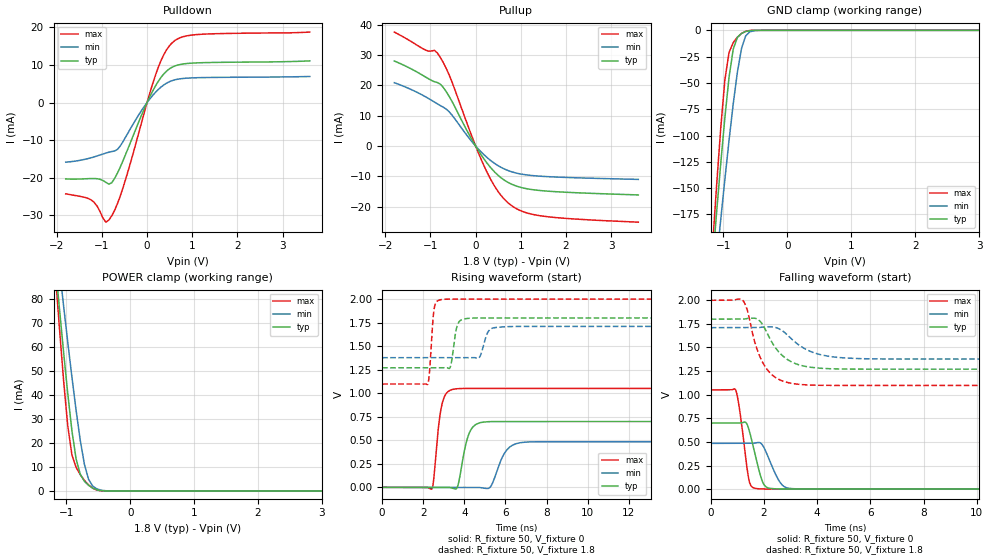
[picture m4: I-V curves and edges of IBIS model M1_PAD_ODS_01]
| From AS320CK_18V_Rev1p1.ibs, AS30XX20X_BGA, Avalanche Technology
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[Model] M1_PAD_ODS_01
Model_type I/O
Enable   Active-High
Vinl  =  0.63
Vinh  =  1.17
Vmeas =  0.9
Cref  =  30e-12
| Capacitance  typ   min   max
C_comp   1.624629e-12   1.520611e-12   1.744819e-12
| Variables   typ   min   max
[GND Clamp Reference]   0   0   0
[POWER Clamp Reference]   1.8   1.71   2
[Pulldown Reference]   0   0   0
[Pullup Reference]   1.8   1.71   2
[Temperature Range]   25   125   -40
[Voltage Range]   1.8   1.71   2
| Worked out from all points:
|   slope of the pulldown table from 0 to 0.27 V, typ, clamps not added: 44.9 ohm
|   slope of the pullup table from 0 to 0.27 V, typ, clamps not added: 45.3 ohm
|   GND clamp passes 1 mA (typ) near -0.64 V on its own axis
|   POWER clamp passes 1 mA (typ) near -0.57 V on its own axis
|   falling waveform, R_fixture 50, V_fixture 0: 20-80 % time 369ps typ, 461ps min, 285ps max; typ from 0.7 V to 0 V
|   falling waveform, R_fixture 50, V_fixture 1.8: 20-80 % time 819ps typ, 1.04ns min, 647ps max; typ from 1.8 V to 1.27 V
|   rising waveform, R_fixture 50, V_fixture 0: 20-80 % time 407ps typ, 569ps min, 308ps max; typ from 0 V to 0.7 V
|   rising waveform, R_fixture 50, V_fixture 1.8: 20-80 % time 214ps typ, 282ps min, 165ps max; typ from 1.27 V to 1.8 V
[GND Clamp]
| Voltage   I(typ)   I(min)   I(max)
-1.8V     -720.4mA   -670.5mA   -825.2mA
-1.173V   -222.3mA   -260.3mA   -207.5mA
-1.108V   -173.8mA   -219.8mA   -148.3mA
-1.043V   -126.9mA   -180.1mA   -93.11mA
-977.6mV  -83.02mA   -141.5mA   -47.01mA
-912.4mV  -44.68mA   -104.6mA   -21.04mA
-847.2mV  -17.95mA   -70.1mA    -11.75mA
-782.1mV  -6.736mA   -39.85mA   -6.526mA
-716.9mV  -2.917mA   -17.13mA   -2.96mA
-651.7mV  -1.107mA   -5.246mA   -907.6uA
-456.2mV  -3.886uA   -74.14uA   -373.5nA
3.6V      0A         0A         0A
[POWER Clamp]
| Voltage   I(typ)   I(min)   I(max)
-1.8V     287.1mA    268.3mA    329.6mA
-1.173V   94.89mA    108.5mA    91.02mA
-1.108V   76.1mA     92.66mA    67.97mA
-1.043V   57.9mA     77.16mA    46.14mA
-977.6mV  40.62mA    62.05mA    27.14mA
-912.4mV  25.13mA    47.46mA    15.06mA
-847.2mV  13.38mA    33.64mA    9.853mA
-716.9mV  4.014mA    11.09mA    4.394mA
-651.7mV  2.34mA     4.821mA    2.483mA
-586.6mV  1.18mA     2.003mA    1.113mA
-325.9mV  1.153uA    19.85uA    110.1nA
3.6V      0A         0A         0A
[Pulldown]
| Voltage   I(typ)   I(min)   I(max)
-1.8V     -20.29mA   -15.84mA   -24.25mA
-1.238V   -20.19mA   -14.67mA   -25.87mA
-912.4mV  -21.19mA   -13.43mA   -31.79mA
-847.2mV  -21.68mA   -13.2mA    -31.24mA
-716.9mV  -20.15mA   -12.86mA   -28.61mA
-521.4mV  -15.14mA   -10.15mA   -22.2mA
-65.17mV  -1.742mA   -1.091mA   -2.802mA
248.3mV   5.63mA     3.46mA     9.353mA
434.5mV   8.383mA    5.171mA    14.07mA
620.7mV   9.735mA    6.051mA    16.51mA
1.179V    10.57mA    6.614mA    18.12mA
3.6V      11.06mA    6.923mA    18.71mA
[Pullup]
| Voltage   I(typ)   I(min)   I(max)
-1.8V     28.07mA    20.9mA     37.6mA
-1.108V   22.77mA    16.25mA    31.67mA
-912.4mV  21.23mA    14.53mA    31.58mA
-782.1mV  20.42mA    13.35mA    29.27mA
-586.6mV  16.4mA     11.32mA    23.49mA
-65.17mV  1.669mA    1.14mA     2.505mA
248.3mV   -5.556mA   -3.722mA   -8.519mA
496.6mV   -9.653mA   -6.467mA   -14.99mA
744.8mV   -12.21mA   -8.229mA   -19.08mA
1.055V    -13.85mA   -9.372mA   -21.68mA
1.49V     -14.76mA   -10.01mA   -23.13mA
3.6V      -16.13mA   -11mA      -25.12mA
[Ramp]
dV/dt_r   0.419845/0.40709n  0.290904/0.569117n  0.630672/0.308383n
dV/dt_f   0.317972/0.818691n  0.199636/1.04487n  0.541445/0.646878n
R_load = 50
[Falling Waveform]
R_fixture = 50
V_fixture = 0
V_fixture_min = 0
V_fixture_max = 0
| Time   V(typ)   V(min)   V(max)
0s        699.7mV    484.8mV    1.051V
936.6ps   700.2mV    485.3mV    1.051V
1.089ns   700.3mV    485.4mV    839.3mV
1.43ns    639mV      485.6mV    108.6mV
1.732ns   294.8mV    491.4mV    6.152mV
1.952ns   76.13mV    465.2mV    2.032mV
2.096ns   21.34mV    384.1mV    1.262mV
2.616ns   1.831mV    69mV       474.1uV
3.058ns   724uV      5.937mV    463.2uV
21.88ns   1.404nV    117.1nV    -317.4nV
[Falling Waveform]
R_fixture = 50
V_fixture = 1.8
V_fixture_min = 1.71
V_fixture_max = 2
| Time   V(typ)   V(min)   V(max)
0s        1.8V       1.71V      2V
1.173ns   1.801V     1.71V      2.008V
1.362ns   1.807V     1.711V     1.909V
1.709ns   1.807V     1.711V     1.511V
2.045ns   1.695V     1.717V     1.297V
2.543ns   1.458V     1.701V     1.165V
3.19ns    1.329V     1.553V     1.114V
4.145ns   1.28V      1.423V     1.1V
5.594ns   1.271V     1.382V     1.098V
21.88ns   1.27V      1.377V     1.098V
[Rising Waveform]
R_fixture = 50
V_fixture = 0
V_fixture_min = 0
V_fixture_max = 0
| Time   V(typ)   V(min)   V(max)
0s        2.363nV    66.36nV    1.939nV
2.414ns   -364.9uV   -508uV     -18.9mV
2.899ns   -438.2uV   -609.9uV   867.9mV
3.517ns   -14.89mV   -740.1uV   1.045V
3.717ns   42.31mV    -782.1uV   1.049V
4.27ns    590.4mV    -898.5uV   1.05V
4.904ns   692.4mV    -7.095mV   1.05V
6.058ns   699mV      394.8mV    1.05V
6.727ns   699mV      474.1mV    1.05V
21.88ns   699.7mV    484.8mV    1.051V
[Rising Waveform]
R_fixture = 50
V_fixture = 1.8
V_fixture_min = 1.71
V_fixture_max = 2
| Time   V(typ)   V(min)   V(max)
0s        1.27V      1.377V     1.098V
2.212ns   1.271V     1.378V     1.092V
2.54ns    1.271V     1.378V     1.907V
2.88ns    1.271V     1.378V     1.994V
3.308ns   1.272V     1.378V     1.999V
3.649ns   1.714V     1.378V     1.999V
4.093ns   1.793V     1.378V     1.999V
4.72ns    1.799V     1.377V     1.999V
5.677ns   1.799V     1.701V     1.999V
21.88ns   1.8V       1.71V      2V
